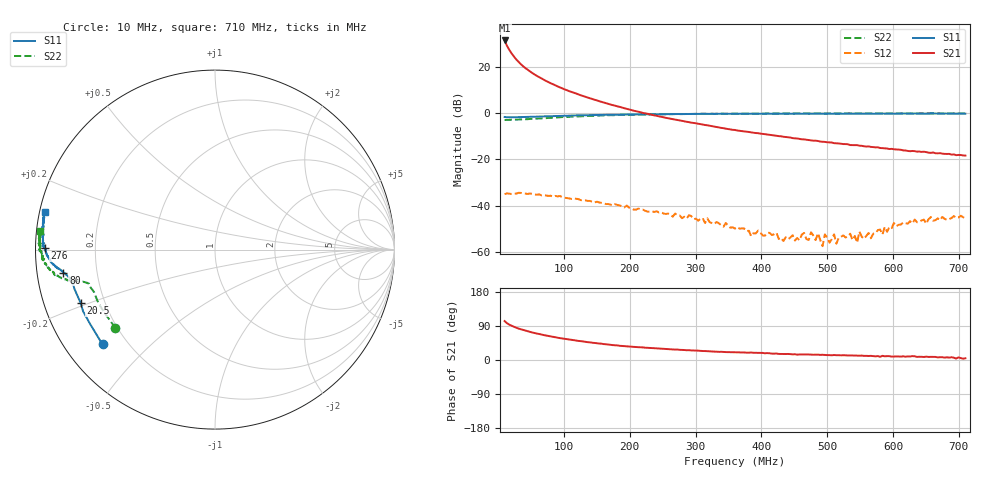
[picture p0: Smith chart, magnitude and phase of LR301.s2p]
!  POLYFET RF DEVICES
!  LR301 (Each Side)
!  S PARAMETERS
!  VDS=28V, IDQ=400mA
! Date: Wed Mar 05 14:34:01 2003
# MHZ S MA R 50
! Freq=Mhz Mag[s11] Ang[s11] Mag[s21] Ang[s21] Mag[s12] Ang[s12] Mag[s22] Ang[s22]
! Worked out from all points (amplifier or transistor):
!   201 points, 10 MHz to 710 MHz, reference 50 ohm
!   highest |S21| = 31.3 dB at 10 MHz (marker M1)
!   |S21| within 3 dB of that: start of sweep to 15 MHz
!   unconditionally stable (mu >= 1): 350.9 MHz to 360.8 MHz; 376.3 MHz to 408.1 MHz; 412.6 MHz to end of sweep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
!   at 125.5 MHz: K = 0.19, MSG = 22.6 dB, |S12| = -37.6 dB
!   at 360 MHz: K = 1.04, MAG = 20.1 dB, |S12| = -50.0 dB
!   at 710 MHz: K = 2.22, MAG = 7.3 dB, |S12| = -45.5 dB
!   S11 on the Smith chart (normalised r, x): 10 MHz: 0.11, -0.36; 20.5 MHz: 0.11, -0.19; 80 MHz: 0.08, -0.07; 276 MHz: 0.03, +0.00; 710 MHz: 0.02, +0.11
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10  0.8198 -139.8  36.84 102.8  0.0177 12.8  0.7058 -141.9
13.5  0.8101 -149.4  28.42 97.3  0.01834 7.9  0.7097 -150.3
17  0.8113 -154.9  23.27 93.3  0.01815 4.1  0.7145 -155.2
20.5  0.8055 -158.4  19.46 90.4  0.01787 2.5  0.7142 -158.4
24  0.8078 -161.0  16.67 87.8  0.01834 -1.1  0.7141 -160.5
27.5  0.8113 -163.1  14.44 85.4  0.01807 -5.0  0.7193 -162.0
31  0.8133 -164.5  12.76 83.0  0.01884 -6.4  0.7246 -163.0
34.5  0.8132 -166.0  11.37 81.2  0.01881 -8.0  0.7264 -164.1
41.5  0.818 -167.7  9.341 77.4  0.0181 -9.4  0.7327 -165.1
48.5  0.8213 -168.7  7.878 74.3  0.01825 -12.6  0.7441 -165.7
59  0.8327 -169.8  6.324 69.7  0.01717 -16.8  0.7577 -166.4
80  0.8546 -171.4  4.384 62.3  0.01636 -23.2  0.7868 -167.0
101  0.8692 -172.7  3.239 55.9  0.01481 -27.0  0.8196 -167.7
129  0.8916 -174.0  2.326 49.0  0.01296 -35.5  0.851 -168.8
174.5  0.9184 -175.9  1.481 39.2  0.01004 -41.1  0.8952 -171.0
244.5  0.9414 -179.0  0.8445 30.4  0.00711 -41.5  0.9363 -173.8
276  0.9499 179.5  0.6924 26.9  0.00611 -38.5  0.9452 -175.0
360  0.9607 176.9  0.4298 20.7  0.00318 -41.4  0.9655 -178.1
479  0.9705 173.3  0.252 13.9  0.00226 16.7  0.9755 178.5
545.5  0.97 171.4  0.2018 11.7  0.00159 49.5  0.9822 177.0
594.5  0.9683 170.1  0.1666 10.1  0.00346 77.7  0.977 176.0
710  0.9675 167.5  0.1202 4.6  0.00529 90.5  0.9816 173.8
